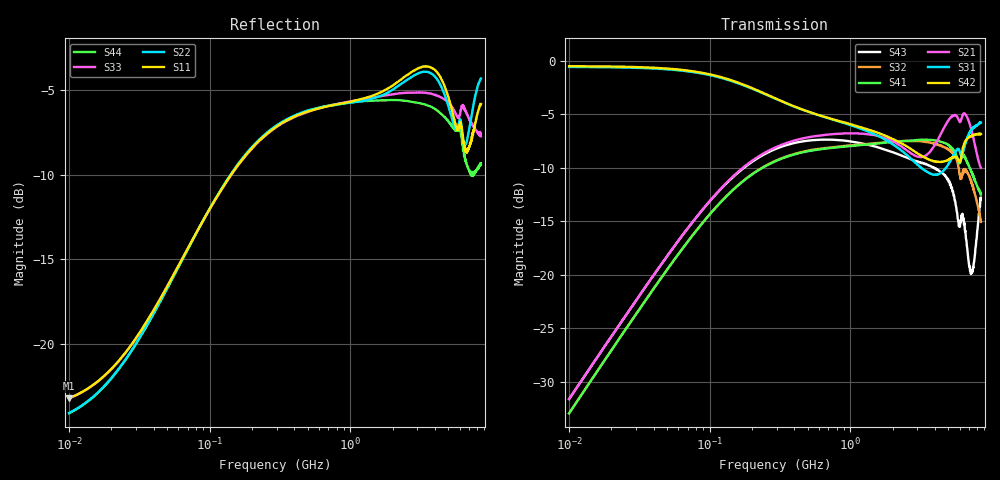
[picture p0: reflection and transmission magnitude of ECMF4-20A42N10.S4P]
!ECMF4-20A42N10
! P1: D1+ or D2+ IN  -ccccc-  P3: D1+ or D2+ OUT
! P2: D1- or D2- IN  -ccccc-  P4: D1- or D2- OUT
!Typical device
!Probes on bumps or pads
!P1 Probe Type :ACP40-GSS-400; Probe S/N : 9H27Q-1
!P2 Probe Type :ACP40-GSS-400; Probe S/N : 9H27Q-1
!P3 Probe Type :ACP40-SSG-400; Probe S/N : DP27Z
!P4 Probe Type :ACP40-SSG-400; Probe S/N : DP27Z
!Instrument Manufacturer: Agilent Technologies
!Instrument Model: E5071B
!Instrument Serial Number: MY42301810
!Instrument Firmware Rev: A.09.10
!Start Freq. :10.000MHz; Stop Freq. : 8.500GHz
!Number of points : 1601; Sweep : LOGARITHMIC
!Ports power : 0.000000dBm; IFBW : 100.000000Hz
!Calibration kit : 129-248 (9090)
!Prober : PM8 (Manual prober)
!Darkness measurement :NO
!Voltage measurement :NO
!Temperature measurement :NO
# Hz S dB R 50
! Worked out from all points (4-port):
!   1601 points, 10 MHz to 8.5 GHz, reference 50 ohm
!   strongest paths, dB at 10 MHz, 54.53 MHz, 295.3 MHz, 1.588 GHz, 8.5 GHz:
!     S42: -0.5, -0.8, -3.5, -6.8, -6.9
!     S31: -0.6, -0.8, -3.6, -7.0, -5.8
!     S21: -31.6, -17.5, -8.1, -7.0, -10.0
!     S41: -32.9, -18.8, -9.4, -7.7, -12.5
!     S32: -32.9, -18.8, -9.3, -7.7, -15.0
!     S43: -31.6, -17.5, -8.2, -8.1, -12.8
!   lowest |S11| = -23.2 dB at 10 MHz (marker M1), VSWR 1.15, Z = 56.8 + j2.82 ohm
!   |S11| at or under -10 dB: start of sweep to 142 MHz
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1e7  -23.19 20.9  -31.59 85.0  -0.58 -1.8  -32.93 -95.1
     -31.59 85.0  -24.07 24.0  -32.92 -95.2  -0.51 -1.8
     -0.58 -1.8  -32.91 -95.1  -23.21 20.7  -31.58 84.9
     -32.92 -95.2  -0.51 -1.9  -31.59 84.8  -24.09 23.8
1.303197e8  -10.46 44.4  -11.44 53.9  -1.72 -18.7  -12.71 -132.1
            -11.45 53.7  -10.43 45.7  -12.72 -132.2  -1.66 -19.1
            -1.73 -18.7  -12.70 -132.1  -10.49 42.5  -11.49 52.2
            -12.71 -132.3  -1.66 -19.2  -11.50 52.1  -10.45 44.0
6.84583e8  -5.97 12.8  -6.83 12.2  -5.35 -37.9  -8.17 162.5
           -6.90 12.5  -5.96 12.4  -8.18 161.9  -5.32 -39.1
           -5.34 -37.9  -8.13 161.9  -5.96 2.5  -7.30 6.6
           -8.19 162.3  -5.32 -39.1  -7.37 6.9  -5.94 3.2
2.103348e9  -4.61 0.4  -7.65 -6.8  -8.04 -86.3  -7.62 92.4
            -7.67 -4.5  -4.87 1.1  -7.52 91.4  -7.49 -87.6
            -7.99 -86.6  -7.54 91.0  -5.23 -33.3  -8.69 -13.4
            -7.55 92.4  -7.44 -87.8  -8.63 -11.2  -5.60 -30.2
4.139176e9  -3.94 -28.9  -7.75 11.2  -11.01 -177.3  -7.81 24.5
            -7.52 12.2  -4.37 -25.3  -7.60 23.5  -9.78 -169.3
            -10.64 -178.9  -7.82 22.2  -5.33 -79.7  -10.65 -18.6
            -7.48 23.1  -9.45 -170.7  -10.13 -18.2  -6.21 -70.9
7.394018e9  -7.74 -29.1  -6.91 -31.7  -6.79 58.6  -9.51 -74.6
            -6.80 -26.5  -6.24 -18.8  -10.66 -71.5  -6.93 69.4
            -6.40 53.7  -11.69 -66.3  -7.05 -146.8  -21.87 12.7
            -10.67 -78.1  -7.02 63.4  -19.59 16.6  -9.86 -122.6
8.5e9  -5.83 -39.6  -11.13 -24.4  -5.90 24.6  -11.78 -120.2
       -9.99 -17.8  -4.33 -34.3  -13.21 -115.6  -6.54 33.4
       -5.77 20.6  -15.04 -104.8  -7.74 -162.8  -14.00 56.9
       -12.50 -125.3  -6.86 28.3  -12.79 47.9  -9.33 -133.3
